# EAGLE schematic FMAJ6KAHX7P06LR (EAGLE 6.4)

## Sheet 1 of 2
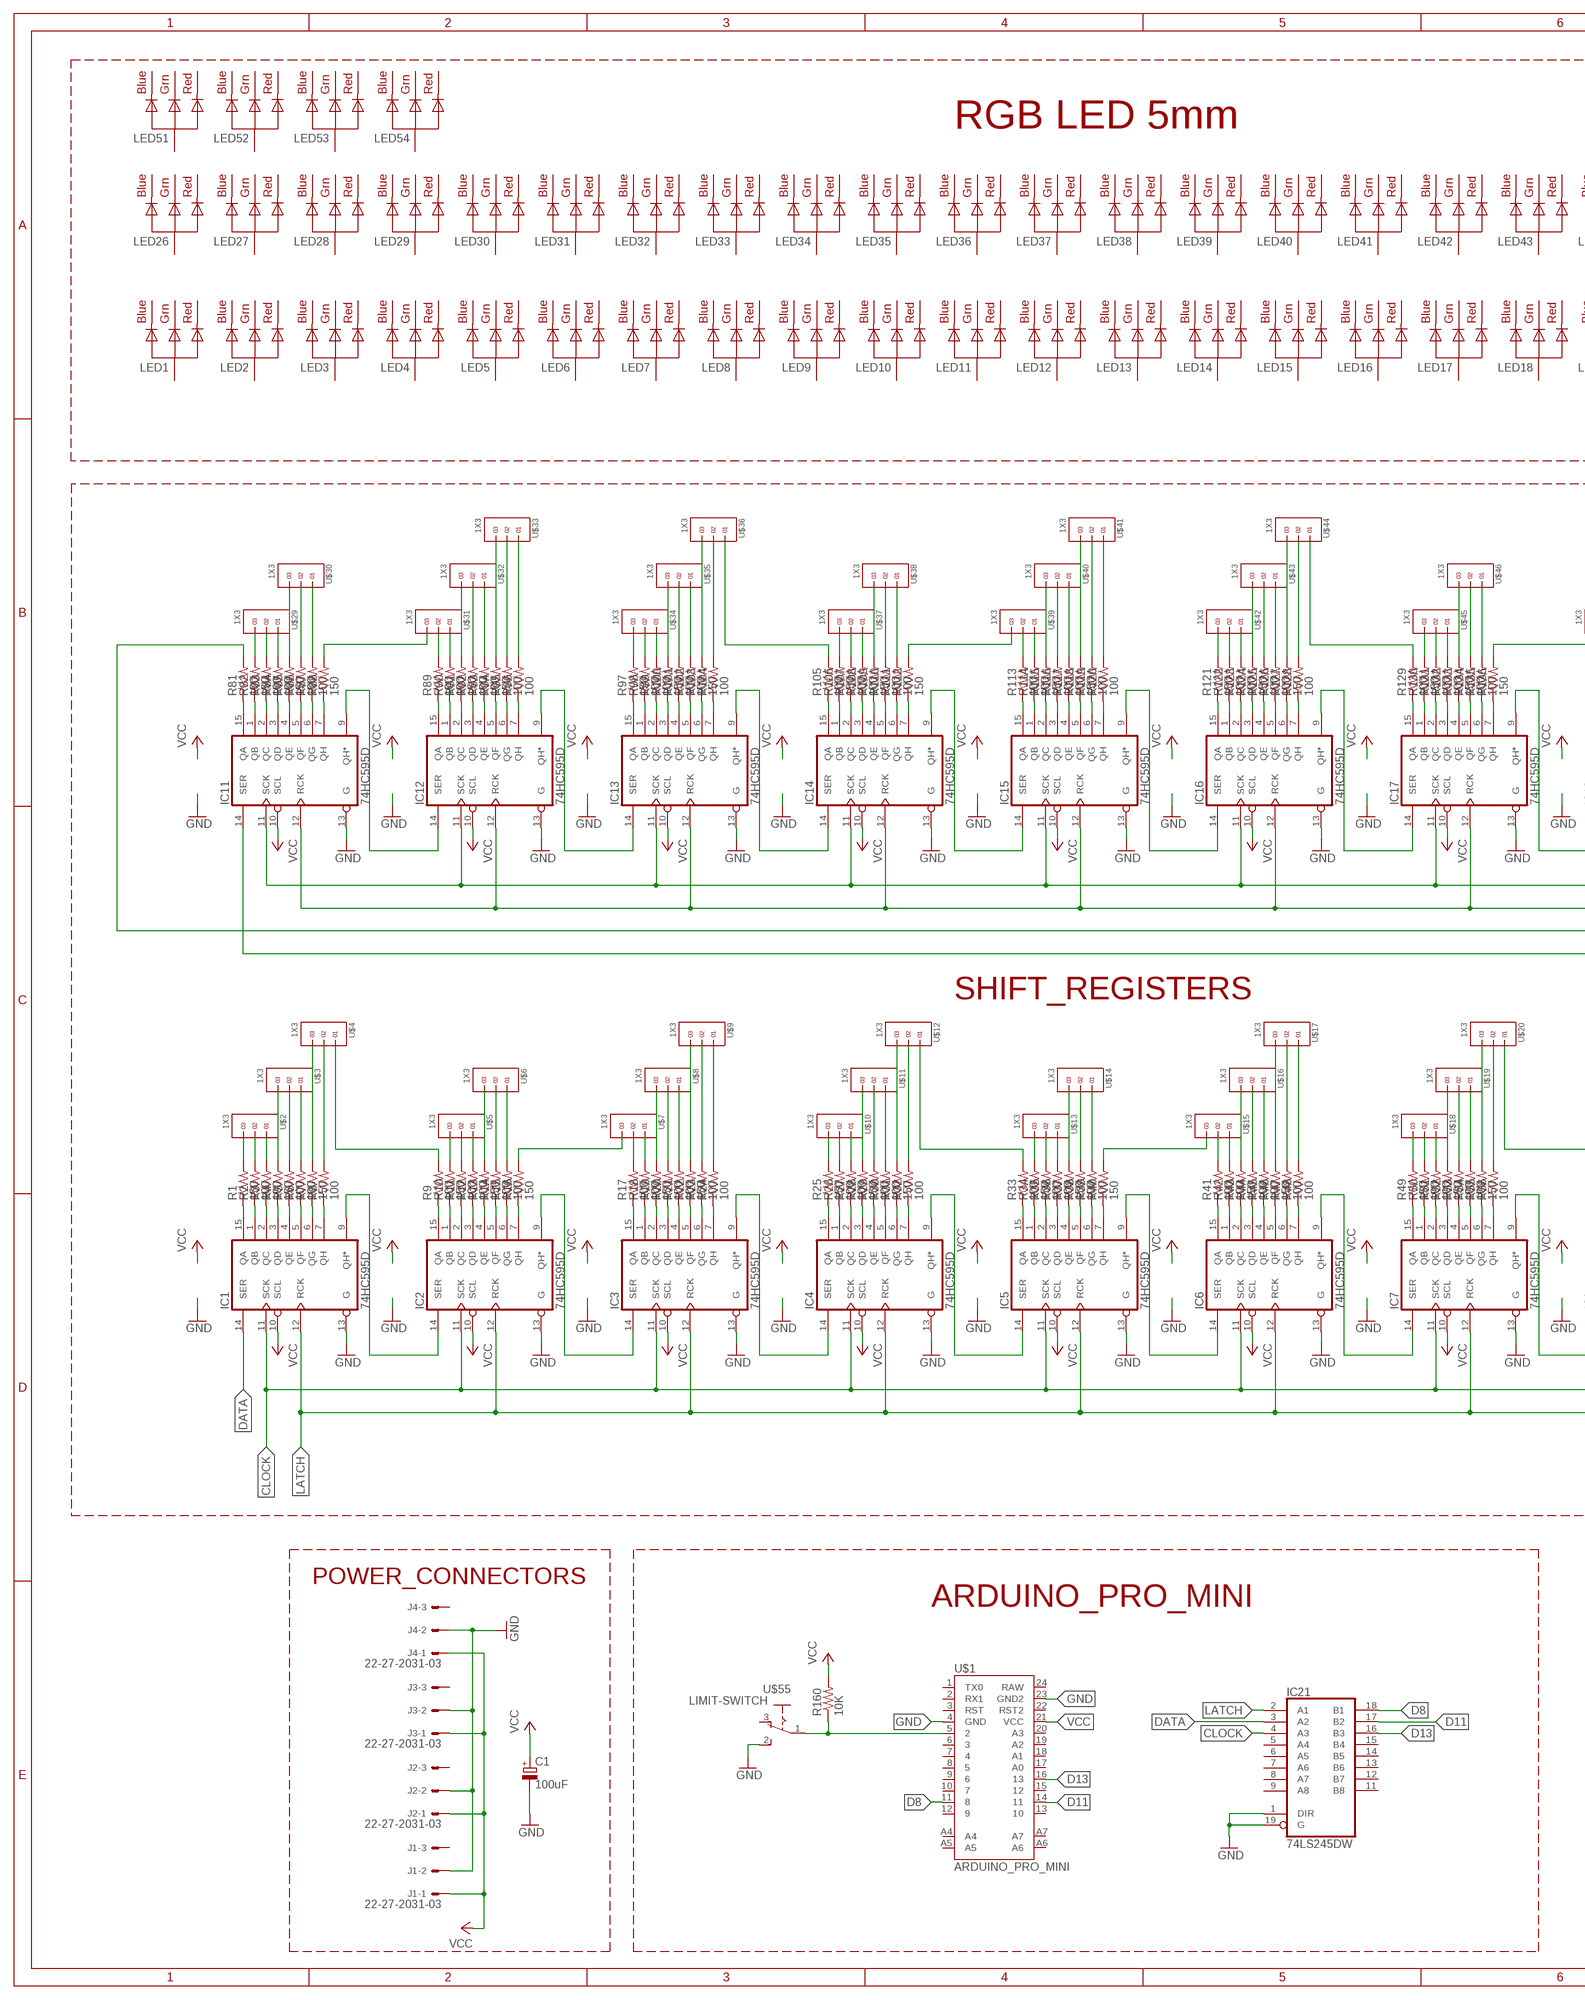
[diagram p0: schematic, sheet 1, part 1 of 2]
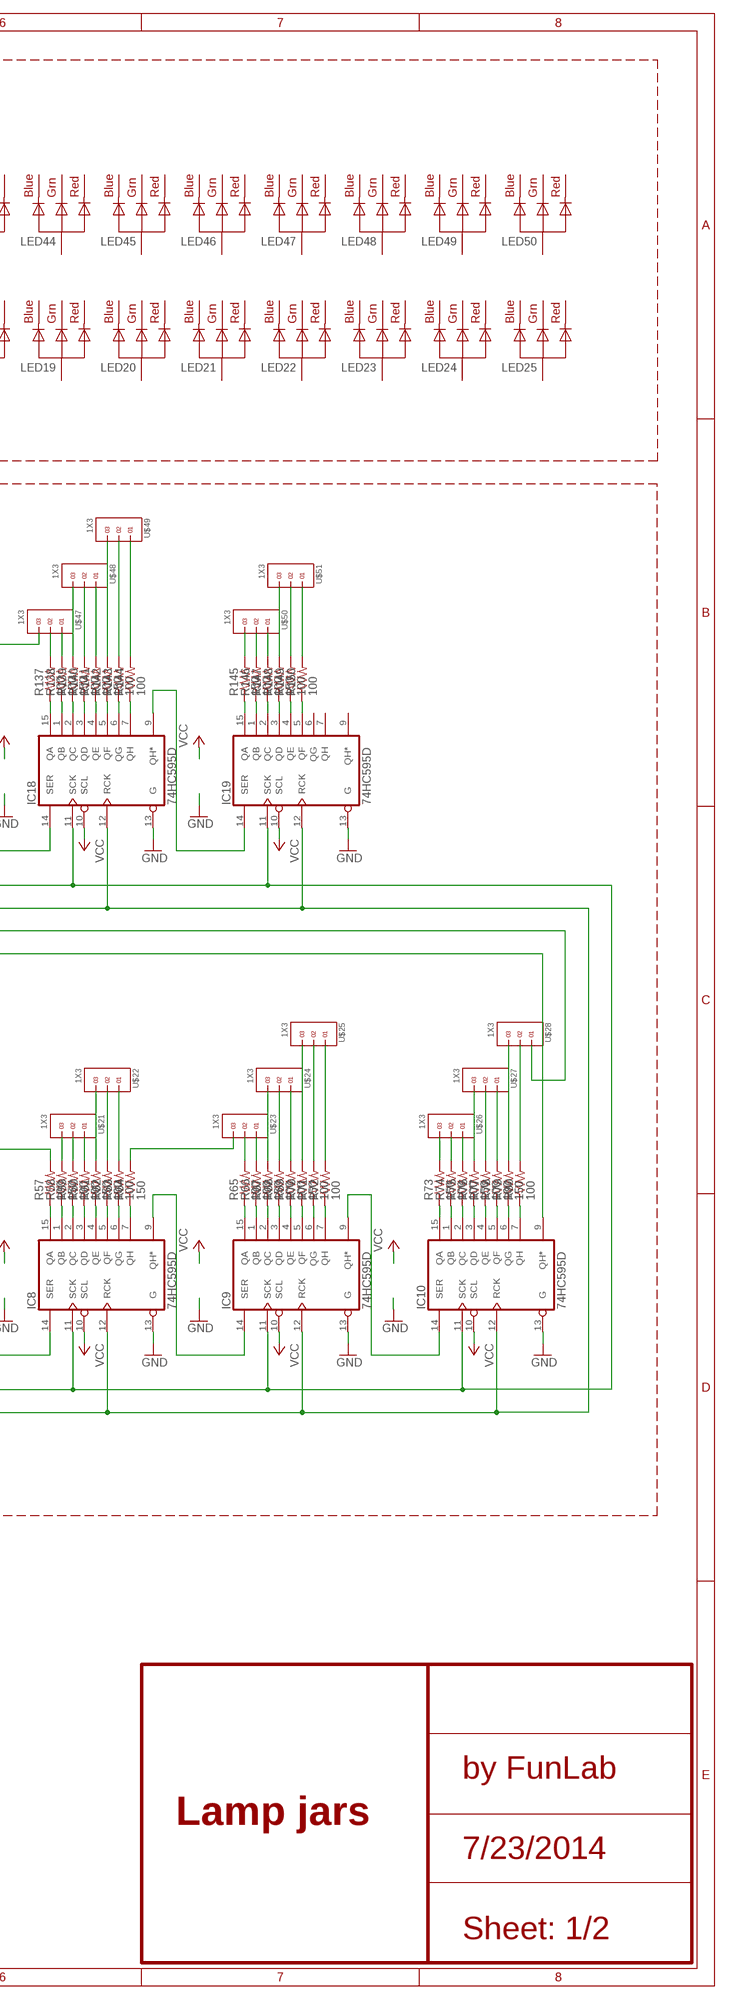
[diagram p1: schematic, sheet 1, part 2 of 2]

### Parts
C1  100uF  CPOL-EUE2.5-6  [E2,5-6]
IC1  74HC595D  [SO16]
IC2  74HC595D  [SO16]
IC3  74HC595D  [SO16]
IC4  74HC595D  [SO16]
IC5  74HC595D  [SO16]
IC6  74HC595D  [SO16]
IC7  74HC595D  [SO16]
IC8  74HC595D  [SO16]
IC9  74HC595D  [SO16]
IC10  74HC595D  [SO16]
IC11  74HC595D  [SO16]
IC12  74HC595D  [SO16]
IC13  74HC595D  [SO16]
IC14  74HC595D  [SO16]
IC15  74HC595D  [SO16]
IC16  74HC595D  [SO16]
IC17  74HC595D  [SO16]
IC18  74HC595D  [SO16]
IC19  74HC595D  [SO16]
IC21  74LS245DW  [SO20W]
J1  22-27-2031-03  [6410-03]
J2  22-27-2031-03  [6410-03]
J3  22-27-2031-03  [6410-03]
J4  22-27-2031-03  [6410-03]
LED1  RGBLED_CA-5MM  [LED5MMRGB]
LED2  RGBLED_CA-5MM  [LED5MMRGB]
LED3  RGBLED_CA-5MM  [LED5MMRGB]
LED4  RGBLED_CA-5MM  [LED5MMRGB]
LED5  RGBLED_CA-5MM  [LED5MMRGB]
LED6  RGBLED_CA-5MM  [LED5MMRGB]
LED7  RGBLED_CA-5MM  [LED5MMRGB]
LED8  RGBLED_CA-5MM  [LED5MMRGB]
LED9  RGBLED_CA-5MM  [LED5MMRGB]
LED10  RGBLED_CA-5MM  [LED5MMRGB]
LED11  RGBLED_CA-5MM  [LED5MMRGB]
LED12  RGBLED_CA-5MM  [LED5MMRGB]
LED13  RGBLED_CA-5MM  [LED5MMRGB]
LED14  RGBLED_CA-5MM  [LED5MMRGB]
LED15  RGBLED_CA-5MM  [LED5MMRGB]
LED16  RGBLED_CA-5MM  [LED5MMRGB]
LED17  RGBLED_CA-5MM  [LED5MMRGB]
LED18  RGBLED_CA-5MM  [LED5MMRGB]
LED19  RGBLED_CA-5MM  [LED5MMRGB]
LED20  RGBLED_CA-5MM  [LED5MMRGB]
LED21  RGBLED_CA-5MM  [LED5MMRGB]
LED22  RGBLED_CA-5MM  [LED5MMRGB]
LED23  RGBLED_CA-5MM  [LED5MMRGB]
LED24  RGBLED_CA-5MM  [LED5MMRGB]
LED25  RGBLED_CA-5MM  [LED5MMRGB]
LED26  RGBLED_CA-5MM  [LED5MMRGB]
LED27  RGBLED_CA-5MM  [LED5MMRGB]
LED28  RGBLED_CA-5MM  [LED5MMRGB]
LED29  RGBLED_CA-5MM  [LED5MMRGB]
LED30  RGBLED_CA-5MM  [LED5MMRGB]
LED31  RGBLED_CA-5MM  [LED5MMRGB]
LED32  RGBLED_CA-5MM  [LED5MMRGB]
LED33  RGBLED_CA-5MM  [LED5MMRGB]
LED34  RGBLED_CA-5MM  [LED5MMRGB]
LED35  RGBLED_CA-5MM  [LED5MMRGB]
LED36  RGBLED_CA-5MM  [LED5MMRGB]
LED37  RGBLED_CA-5MM  [LED5MMRGB]
LED38  RGBLED_CA-5MM  [LED5MMRGB]
LED39  RGBLED_CA-5MM  [LED5MMRGB]
LED40  RGBLED_CA-5MM  [LED5MMRGB]
LED41  RGBLED_CA-5MM  [LED5MMRGB]
LED42  RGBLED_CA-5MM  [LED5MMRGB]
LED43  RGBLED_CA-5MM  [LED5MMRGB]
LED44  RGBLED_CA-5MM  [LED5MMRGB]
LED45  RGBLED_CA-5MM  [LED5MMRGB]
LED46  RGBLED_CA-5MM  [LED5MMRGB]
LED47  RGBLED_CA-5MM  [LED5MMRGB]
LED48  RGBLED_CA-5MM  [LED5MMRGB]
LED49  RGBLED_CA-5MM  [LED5MMRGB]
LED50  RGBLED_CA-5MM  [LED5MMRGB]
LED51  RGBLED_CA-5MM  [LED5MMRGB]
LED52  RGBLED_CA-5MM  [LED5MMRGB]
LED53  RGBLED_CA-5MM  [LED5MMRGB]
LED54  RGBLED_CA-5MM  [LED5MMRGB]
R1  150  R-US_M0805  [M0805]
R2  100  R-US_M0805  [M0805]
R3  100  R-US_M0805  [M0805]
R4  150  R-US_M0805  [M0805]
R5  100  R-US_M0805  [M0805]
R6  100  R-US_M0805  [M0805]
R7  150  R-US_M0805  [M0805]
R8  100  R-US_M0805  [M0805]
R9  100  R-US_M0805  [M0805]
R10  150  R-US_M0805  [M0805]
R11  100  R-US_M0805  [M0805]
R12  100  R-US_M0805  [M0805]
R13  150  R-US_M0805  [M0805]
R14  100  R-US_M0805  [M0805]
R15  100  R-US_M0805  [M0805]
R16  150  R-US_M0805  [M0805]
R17  100  R-US_M0805  [M0805]
R18  100  R-US_M0805  [M0805]
R19  150  R-US_M0805  [M0805]
R20  100  R-US_M0805  [M0805]
R21  100  R-US_M0805  [M0805]
R22  150  R-US_M0805  [M0805]
R23  100  R-US_M0805  [M0805]
R24  100  R-US_M0805  [M0805]
R25  150  R-US_M0805  [M0805]
R26  100  R-US_M0805  [M0805]
R27  100  R-US_M0805  [M0805]
R28  150  R-US_M0805  [M0805]
R29  100  R-US_M0805  [M0805]
R30  100  R-US_M0805  [M0805]
R31  150  R-US_M0805  [M0805]
R32  100  R-US_M0805  [M0805]
R33  100  R-US_M0805  [M0805]
R34  150  R-US_M0805  [M0805]
R35  100  R-US_M0805  [M0805]
R36  100  R-US_M0805  [M0805]
R37  150  R-US_M0805  [M0805]
R38  100  R-US_M0805  [M0805]
R39  100  R-US_M0805  [M0805]
R40  150  R-US_M0805  [M0805]
R41  100  R-US_M0805  [M0805]
R42  100  R-US_M0805  [M0805]
R43  150  R-US_M0805  [M0805]
R44  100  R-US_M0805  [M0805]
R45  100  R-US_M0805  [M0805]
R46  150  R-US_M0805  [M0805]
R47  100  R-US_M0805  [M0805]
R48  100  R-US_M0805  [M0805]
R49  150  R-US_M0805  [M0805]
R50  100  R-US_M0805  [M0805]
R51  100  R-US_M0805  [M0805]
R52  150  R-US_M0805  [M0805]
R53  100  R-US_M0805  [M0805]
R54  100  R-US_M0805  [M0805]
R55  150  R-US_M0805  [M0805]
R56  100  R-US_M0805  [M0805]
R57  100  R-US_M0805  [M0805]
R58  150  R-US_M0805  [M0805]
R59  100  R-US_M0805  [M0805]
R60  100  R-US_M0805  [M0805]
R61  150  R-US_M0805  [M0805]
R62  100  R-US_M0805  [M0805]
R63  100  R-US_M0805  [M0805]
R64  150  R-US_M0805  [M0805]
R65  100  R-US_M0805  [M0805]
R66  100  R-US_M0805  [M0805]
R67  150  R-US_M0805  [M0805]
R68  100  R-US_M0805  [M0805]
R69  100  R-US_M0805  [M0805]
R70  150  R-US_M0805  [M0805]
R71  100  R-US_M0805  [M0805]
R72  100  R-US_M0805  [M0805]
R73  150  R-US_M0805  [M0805]
R74  100  R-US_M0805  [M0805]
R75  100  R-US_M0805  [M0805]
R76  150  R-US_M0805  [M0805]
R77  100  R-US_M0805  [M0805]
R78  100  R-US_M0805  [M0805]
R79  150  R-US_M0805  [M0805]
R80  100  R-US_M0805  [M0805]
R81  100  R-US_M0805  [M0805]
R82  150  R-US_M0805  [M0805]
R83  100  R-US_M0805  [M0805]
R84  100  R-US_M0805  [M0805]
R85  150  R-US_M0805  [M0805]
R86  100  R-US_M0805  [M0805]
R87  100  R-US_M0805  [M0805]
R88  150  R-US_M0805  [M0805]
R89  100  R-US_M0805  [M0805]
R90  100  R-US_M0805  [M0805]
R91  150  R-US_M0805  [M0805]
R92  100  R-US_M0805  [M0805]
R93  100  R-US_M0805  [M0805]
R94  150  R-US_M0805  [M0805]
R95  100  R-US_M0805  [M0805]
R96  100  R-US_M0805  [M0805]
R97  150  R-US_M0805  [M0805]
R98  100  R-US_M0805  [M0805]
R99  100  R-US_M0805  [M0805]
R100  150  R-US_M0805  [M0805]
R101  100  R-US_M0805  [M0805]
R102  100  R-US_M0805  [M0805]
R103  150  R-US_M0805  [M0805]
R104  100  R-US_M0805  [M0805]
R105  100  R-US_M0805  [M0805]
R106  150  R-US_M0805  [M0805]
R107  100  R-US_M0805  [M0805]
R108  100  R-US_M0805  [M0805]
R109  150  R-US_M0805  [M0805]
R110  100  R-US_M0805  [M0805]
R111  100  R-US_M0805  [M0805]
R112  150  R-US_M0805  [M0805]
R113  100  R-US_M0805  [M0805]
R114  100  R-US_M0805  [M0805]
R115  150  R-US_M0805  [M0805]
R116  100  R-US_M0805  [M0805]
R117  100  R-US_M0805  [M0805]
R118  150  R-US_M0805  [M0805]
R119  100  R-US_M0805  [M0805]
R120  100  R-US_M0805  [M0805]
R121  150  R-US_M0805  [M0805]
R122  100  R-US_M0805  [M0805]
R123  100  R-US_M0805  [M0805]
R124  150  R-US_M0805  [M0805]
R125  100  R-US_M0805  [M0805]
R126  100  R-US_M0805  [M0805]
R127  150  R-US_M0805  [M0805]
R128  100  R-US_M0805  [M0805]
R129  100  R-US_M0805  [M0805]
R130  150  R-US_M0805  [M0805]
R131  100  R-US_M0805  [M0805]
R132  100  R-US_M0805  [M0805]
R133  150  R-US_M0805  [M0805]
R134  100  R-US_M0805  [M0805]
R135  100  R-US_M0805  [M0805]
R136  150  R-US_M0805  [M0805]
R137  100  R-US_M0805  [M0805]
R138  100  R-US_M0805  [M0805]
R139  150  R-US_M0805  [M0805]
R140  100  R-US_M0805  [M0805]
R141  100  R-US_M0805  [M0805]
R142  150  R-US_M0805  [M0805]
R143  100  R-US_M0805  [M0805]
R144  100  R-US_M0805  [M0805]
R145  150  R-US_M0805  [M0805]
R146  100  R-US_M0805  [M0805]
R147  100  R-US_M0805  [M0805]
R148  150  R-US_M0805  [M0805]
R149  100  R-US_M0805  [M0805]
R150  100  R-US_M0805  [M0805]
R160  10K  R-US_0207/10  [0207/10]
U$1  ARDUINO_PRO_MINI  [ARDUINO_PRO_MINI]
U$2  1X3  [1X3]
U$3  1X3  [1X3]
U$4  1X3  [1X3]
U$5  1X3  [1X3]
U$6  1X3  [1X3]
U$7  1X3  [1X3]
U$8  1X3  [1X3]
U$9  1X3  [1X3]
U$10  1X3  [1X3]
U$11  1X3  [1X3]
U$12  1X3  [1X3]
U$13  1X3  [1X3]
U$14  1X3  [1X3]
U$15  1X3  [1X3]
U$16  1X3  [1X3]
U$17  1X3  [1X3]
U$18  1X3  [1X3]
U$19  1X3  [1X3]
U$20  1X3  [1X3]
U$21  1X3  [1X3]
U$22  1X3  [1X3]
U$23  1X3  [1X3]
U$24  1X3  [1X3]
U$25  1X3  [1X3]
U$26  1X3  [1X3]
U$27  1X3  [1X3]
U$28  1X3  [1X3]
U$29  1X3  [1X3]
U$30  1X3  [1X3]
U$31  1X3  [1X3]
U$32  1X3  [1X3]
U$33  1X3  [1X3]
U$34  1X3  [1X3]
U$35  1X3  [1X3]
U$36  1X3  [1X3]
U$37  1X3  [1X3]
U$38  1X3  [1X3]
U$39  1X3  [1X3]
U$40  1X3  [1X3]
U$41  1X3  [1X3]
U$42  1X3  [1X3]
U$43  1X3  [1X3]
U$44  1X3  [1X3]
U$45  1X3  [1X3]
U$46  1X3  [1X3]
U$47  1X3  [1X3]
U$48  1X3  [1X3]
U$49  1X3  [1X3]
U$50  1X3  [1X3]
U$51  1X3  [1X3]
U$55  LIMIT-SWITCH  [LIMIT-SWITCH]

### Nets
CLOCK: IC1.11(SCK) IC2.11(SCK) IC3.11(SCK) IC4.11(SCK) IC5.11(SCK) IC6.11(SCK) IC7.11(SCK) IC8.11(SCK) IC9.11(SCK) IC10.11(SCK) IC11.11(SCK) IC12.11(SCK) IC13.11(SCK) IC14.11(SCK) IC15.11(SCK) IC16.11(SCK) IC17.11(SCK) IC18.11(SCK) IC19.11(SCK) IC21.4(A3)
D8: IC21.18(B1) U$1.11
D11: IC21.17(B2) U$1.14
D13: IC21.16(B3) U$1.16
DATA: IC1.14(SER) IC21.3(A2)
GND: C1.- IC1.13(G) IC2.13(G) IC3.13(G) IC4.13(G) IC5.13(G) IC6.13(G) IC7.13(G) IC8.13(G) IC9.13(G) IC10.13(G) IC11.13(G) IC12.13(G) IC13.13(G) IC14.13(G) IC15.13(G) IC16.13(G) IC17.13(G) IC18.13(G) IC19.13(G) IC21.1(DIR) IC21.19(G) J1.2 J2.2 J3.2 J4.2 U$1.4(GND) U$1.23(GND2) U$55.2(S) ; also sheet 2
LATCH: IC1.12(RCK) IC2.12(RCK) IC3.12(RCK) IC4.12(RCK) IC5.12(RCK) IC6.12(RCK) IC7.12(RCK) IC8.12(RCK) IC9.12(RCK) IC10.12(RCK) IC11.12(RCK) IC12.12(RCK) IC13.12(RCK) IC14.12(RCK) IC15.12(RCK) IC16.12(RCK) IC17.12(RCK) IC18.12(RCK) IC19.12(RCK) IC21.2(A1)
N$1: R160.1 U$1.5 U$55.1(P)
N$5: R81.2 U$28.1
N$6: IC10.9(QH*) IC11.14(SER)
N$29: IC1.15(QA) R1.1
N$30: IC1.1(QB) R2.1
N$31: IC1.2(QC) R3.1
N$32: R1.2 U$2.3
N$33: R2.2 U$2.2
N$34: R3.2 U$2.1
N$35: R4.2 U$3.3
N$36: R5.2 U$3.2
N$37: R6.2 U$3.1
N$38: R7.2 U$4.3
N$39: R8.2 U$4.2
N$40: IC1.3(QD) R4.1
N$41: IC1.4(QE) R5.1
N$42: IC1.5(QF) R6.1
N$43: IC1.6(QG) R7.1
N$44: IC1.7(QH) R8.1
N$45: IC2.15(QA) R9.1
N$46: R9.2 U$4.1
N$47: R10.2 U$5.3
N$48: R11.2 U$5.2
N$49: R12.2 U$5.1
N$50: R13.2 U$6.3
N$51: R14.2 U$6.2
N$52: R15.2 U$6.1
N$53: R16.2 U$7.3
N$54: R17.2 U$7.2
N$55: R18.2 U$7.1
N$56: R19.2 U$8.3
N$57: R20.2 U$8.2
N$58: R21.2 U$8.1
N$59: R22.2 U$9.3
N$60: R23.2 U$9.2
N$61: R24.2 U$9.1
N$62: R25.2 U$10.3
N$63: R26.2 U$10.2
N$64: R27.2 U$10.1
N$65: R28.2 U$11.3
N$66: R29.2 U$11.2
N$67: R30.2 U$11.1
N$68: R31.2 U$12.3
N$69: R32.2 U$12.2
N$70: R33.2 U$12.1
N$71: R34.2 U$13.3
N$72: R35.2 U$13.2
N$73: R36.2 U$13.1
N$74: R37.2 U$14.3
N$75: R38.2 U$14.2
N$76: R39.2 U$14.1
N$77: R40.2 U$15.3
N$78: R41.2 U$15.2
N$79: R42.2 U$15.1
N$80: R43.2 U$16.3
N$81: R44.2 U$16.2
N$82: R45.2 U$16.1
N$83: R46.2 U$17.3
N$84: R47.2 U$17.2
N$85: R48.2 U$17.1
N$86: R49.2 U$18.3
N$87: R50.2 U$18.2
N$88: R51.2 U$18.1
N$89: R52.2 U$19.3
N$90: R53.2 U$19.2
N$91: R54.2 U$19.1
N$92: R55.2 U$20.3
N$93: R56.2 U$20.2
N$94: R57.2 U$20.1
N$95: R58.2 U$21.3
N$96: R59.2 U$21.2
N$97: R60.2 U$21.1
N$98: R61.2 U$22.3
N$99: R62.2 U$22.2
N$100: R63.2 U$22.1
N$101: R64.2 U$23.3
N$102: R65.2 U$23.2
N$103: R66.2 U$23.1
N$104: R67.2 U$24.3
N$105: R68.2 U$24.2
N$106: R69.2 U$24.1
N$107: R70.2 U$25.3
N$108: R71.2 U$25.2
N$109: R72.2 U$25.1
N$110: R73.2 U$26.3
N$111: R74.2 U$26.2
N$112: R75.2 U$26.1
N$113: R76.2 U$27.3
N$114: R77.2 U$27.2
N$115: R78.2 U$27.1
N$116: R79.2 U$28.3
N$117: R80.2 U$28.2
N$118: R82.2 U$29.3
N$119: R83.2 U$29.2
N$120: R84.2 U$29.1
N$121: R85.2 U$30.3
N$122: R86.2 U$30.2
N$123: R87.2 U$30.1
N$124: R88.2 U$31.3
N$125: R89.2 U$31.2
N$126: R90.2 U$31.1
N$127: R91.2 U$32.3
N$128: R92.2 U$32.2
N$129: R93.2 U$32.1
N$130: R94.2 U$33.3
N$131: R95.2 U$33.2
N$132: R96.2 U$33.1
N$133: R97.2 U$34.3
N$134: R98.2 U$34.2
N$135: R99.2 U$34.1
N$136: R100.2 U$35.3
N$137: R101.2 U$35.2
N$138: R102.2 U$35.1
N$139: R103.2 U$36.3
N$140: R104.2 U$36.2
N$141: R105.2 U$36.1
N$142: R106.2 U$37.3
N$143: R107.2 U$37.2
N$144: R108.2 U$37.1
N$145: R109.2 U$38.3
N$146: R110.2 U$38.2
N$147: R111.2 U$38.1
N$148: R112.2 U$39.3
N$149: R113.2 U$39.2
N$150: R114.2 U$39.1
N$151: R115.2 U$40.3
N$152: R116.2 U$40.2
N$153: R117.2 U$40.1
N$154: R118.2 U$41.3
N$155: R119.2 U$41.2
N$156: R120.2 U$41.1
N$157: R121.2 U$42.3
N$158: R122.2 U$42.2
N$159: R123.2 U$42.1
N$160: R124.2 U$43.3
N$161: R125.2 U$43.2
N$162: R126.2 U$43.1
N$163: R127.2 U$44.3
N$164: R128.2 U$44.2
N$165: R129.2 U$44.1
N$166: R130.2 U$45.3
N$167: R131.2 U$45.2
N$168: R132.2 U$45.1
N$169: R133.2 U$46.3
N$170: R134.2 U$46.2
N$171: R135.2 U$46.1
N$172: R136.2 U$47.3
N$173: R137.2 U$47.2
N$174: R138.2 U$47.1
N$175: R139.2 U$48.3
N$176: R140.2 U$48.2
N$177: R141.2 U$48.1
N$178: R142.2 U$49.3
N$179: R143.2 U$49.2
N$180: R144.2 U$49.1
N$181: R145.2 U$50.3
N$182: R146.2 U$50.2
N$183: R147.2 U$50.1
N$184: R148.2 U$51.3
N$185: R149.2 U$51.2
N$186: R150.2 U$51.1
N$196: IC11.15(QA) R81.1
N$197: IC11.1(QB) R82.1
N$198: IC11.2(QC) R83.1
N$199: IC11.3(QD) R84.1
N$200: IC11.4(QE) R85.1
N$201: IC11.5(QF) R86.1
N$202: IC11.6(QG) R87.1
N$203: IC11.7(QH) R88.1
N$204: IC12.15(QA) R89.1
N$205: IC12.1(QB) R90.1
N$206: IC12.2(QC) R91.1
N$207: IC12.3(QD) R92.1
N$208: IC12.4(QE) R93.1
N$209: IC12.5(QF) R94.1
N$210: IC12.6(QG) R95.1
N$211: IC12.7(QH) R96.1
N$212: IC13.15(QA) R97.1
N$213: IC13.1(QB) R98.1
N$214: IC13.2(QC) R99.1
N$215: IC13.3(QD) R100.1
N$216: IC13.4(QE) R101.1
N$217: IC13.5(QF) R102.1
N$218: IC13.6(QG) R103.1
N$219: IC13.7(QH) R104.1
N$220: IC14.15(QA) R105.1
N$221: IC14.1(QB) R106.1
N$222: IC14.2(QC) R107.1
N$223: IC14.3(QD) R108.1
N$224: IC14.4(QE) R109.1
N$225: IC14.5(QF) R110.1
N$226: IC14.6(QG) R111.1
N$227: IC14.7(QH) R112.1
N$228: IC15.15(QA) R113.1
N$229: IC15.1(QB) R114.1
N$230: IC15.2(QC) R115.1
N$231: IC15.3(QD) R116.1
N$232: IC15.4(QE) R117.1
N$233: IC15.5(QF) R118.1
N$234: IC15.6(QG) R119.1
N$235: IC15.7(QH) R120.1
N$236: IC16.15(QA) R121.1
N$237: IC16.1(QB) R122.1
N$238: IC16.2(QC) R123.1
N$239: IC16.3(QD) R124.1
N$240: IC16.4(QE) R125.1
N$241: IC16.5(QF) R126.1
N$242: IC16.6(QG) R127.1
N$243: IC16.7(QH) R128.1
N$244: IC17.15(QA) R129.1
N$245: IC17.1(QB) R130.1
N$246: IC17.2(QC) R131.1
N$247: IC17.3(QD) R132.1
N$248: IC17.4(QE) R133.1
N$249: IC17.5(QF) R134.1
N$250: IC17.6(QG) R135.1
N$251: IC17.7(QH) R136.1
N$252: IC18.15(QA) R137.1
N$253: IC18.1(QB) R138.1
N$254: IC18.2(QC) R139.1
N$255: IC18.3(QD) R140.1
N$256: IC18.4(QE) R141.1
N$257: IC18.5(QF) R142.1
N$258: IC18.6(QG) R143.1
N$259: IC18.7(QH) R144.1
N$260: IC19.15(QA) R145.1
N$261: IC19.1(QB) R146.1
N$262: IC19.2(QC) R147.1
N$263: IC19.3(QD) R148.1
N$264: IC19.4(QE) R149.1
N$265: IC19.5(QF) R150.1
N$276: IC10.7(QH) R80.1
N$277: IC10.6(QG) R79.1
N$278: IC10.5(QF) R78.1
N$279: IC10.4(QE) R77.1
N$280: IC10.3(QD) R76.1
N$281: IC10.2(QC) R75.1
N$282: IC10.1(QB) R74.1
N$283: IC10.15(QA) R73.1
N$284: IC9.7(QH) R72.1
N$285: IC9.6(QG) R71.1
N$286: IC9.5(QF) R70.1
N$287: IC9.4(QE) R69.1
N$288: IC9.3(QD) R68.1
N$289: IC9.2(QC) R67.1
N$290: IC9.1(QB) R66.1
N$291: IC9.15(QA) R65.1
N$292: IC8.7(QH) R64.1
N$293: IC8.6(QG) R63.1
N$294: IC8.5(QF) R62.1
N$295: IC8.4(QE) R61.1
N$296: IC8.3(QD) R60.1
N$297: IC8.2(QC) R59.1
N$298: IC8.1(QB) R58.1
N$299: IC8.15(QA) R57.1
N$300: IC7.7(QH) R56.1
N$301: IC7.6(QG) R55.1
N$302: IC7.5(QF) R54.1
N$303: IC7.4(QE) R53.1
N$304: IC7.3(QD) R52.1
N$305: IC7.2(QC) R51.1
N$306: IC7.1(QB) R50.1
N$307: IC7.15(QA) R49.1
N$308: IC6.7(QH) R48.1
N$309: IC6.6(QG) R47.1
N$310: IC6.5(QF) R46.1
N$311: IC6.4(QE) R45.1
N$312: IC6.3(QD) R44.1
N$313: IC6.2(QC) R43.1
N$314: IC6.1(QB) R42.1
N$315: IC6.15(QA) R41.1
N$316: IC5.7(QH) R40.1
N$317: IC5.6(QG) R39.1
N$318: IC5.5(QF) R38.1
N$319: IC5.4(QE) R37.1
N$320: IC5.3(QD) R36.1
N$321: IC5.2(QC) R35.1
N$322: IC5.1(QB) R34.1
N$323: IC5.15(QA) R33.1
N$324: IC4.7(QH) R32.1
N$325: IC4.6(QG) R31.1
N$326: IC4.5(QF) R30.1
N$327: IC4.4(QE) R29.1
N$328: IC4.3(QD) R28.1
N$329: IC4.2(QC) R27.1
N$330: IC4.1(QB) R26.1
N$331: IC4.15(QA) R25.1
N$332: IC3.7(QH) R24.1
N$333: IC3.6(QG) R23.1
N$334: IC3.5(QF) R22.1
N$335: IC3.4(QE) R21.1
N$336: IC3.3(QD) R20.1
N$337: IC3.2(QC) R19.1
N$338: IC3.1(QB) R18.1
N$339: IC3.15(QA) R17.1
N$340: IC2.7(QH) R16.1
N$341: IC2.6(QG) R15.1
N$342: IC2.5(QF) R14.1
N$343: IC2.4(QE) R13.1
N$344: IC2.3(QD) R12.1
N$345: IC2.2(QC) R11.1
N$346: IC2.1(QB) R10.1
N$347: IC2.9(QH*) IC3.14(SER)
N$348: IC1.9(QH*) IC2.14(SER)
N$349: IC3.9(QH*) IC4.14(SER)
N$350: IC4.9(QH*) IC5.14(SER)
N$351: IC5.9(QH*) IC6.14(SER)
N$352: IC6.9(QH*) IC7.14(SER)
N$353: IC7.9(QH*) IC8.14(SER)
N$354: IC8.9(QH*) IC9.14(SER)
N$355: IC9.9(QH*) IC10.14(SER)
N$356: IC11.9(QH*) IC12.14(SER)
N$357: IC12.9(QH*) IC13.14(SER)
N$358: IC13.9(QH*) IC14.14(SER)
N$359: IC14.9(QH*) IC15.14(SER)
N$360: IC15.9(QH*) IC16.14(SER)
N$361: IC16.9(QH*) IC17.14(SER)
N$362: IC17.9(QH*) IC18.14(SER)
N$363: IC18.9(QH*) IC19.14(SER)
VCC: C1.+ IC1.10(SCL) IC2.10(SCL) IC3.10(SCL) IC4.10(SCL) IC5.10(SCL) IC6.10(SCL) IC7.10(SCL) IC8.10(SCL) IC9.10(SCL) IC10.10(SCL) IC11.10(SCL) IC12.10(SCL) IC13.10(SCL) IC14.10(SCL) IC15.10(SCL) IC16.10(SCL) IC17.10(SCL) IC18.10(SCL) IC19.10(SCL) J1.1 J2.1 J3.1 J4.1 R160.2 U$1.21(VCC) ; also sheet 2
Unconnected: IC19.6(QG) IC19.7(QH) IC19.9(QH*) IC21.5(A4) IC21.6(A5) IC21.7(A6) IC21.8(A7) IC21.9(A8) IC21.11(B8) IC21.12(B7) IC21.13(B6) IC21.14(B5) IC21.15(B4) J1.3 J2.3 J3.3 J4.3 LED1.1(RED) LED1.2(VCC) LED1.3(GREEN) LED1.4(BLUE) LED2.1(RED) LED2.2(VCC) LED2.3(GREEN) LED2.4(BLUE) LED3.1(RED) LED3.2(VCC) LED3.3(GREEN) LED3.4(BLUE) LED4.1(RED) LED4.2(VCC) LED4.3(GREEN) LED4.4(BLUE) LED5.1(RED) LED5.2(VCC) LED5.3(GREEN) LED5.4(BLUE) LED6.1(RED) LED6.2(VCC) LED6.3(GREEN) LED6.4(BLUE) LED7.1(RED) LED7.2(VCC) LED7.3(GREEN) LED7.4(BLUE) LED8.1(RED) LED8.2(VCC) LED8.3(GREEN) LED8.4(BLUE) LED9.1(RED) LED9.2(VCC) LED9.3(GREEN) LED9.4(BLUE) LED10.1(RED) LED10.2(VCC) LED10.3(GREEN) LED10.4(BLUE) LED11.1(RED) LED11.2(VCC) LED11.3(GREEN) LED11.4(BLUE) LED12.1(RED) LED12.2(VCC) LED12.3(GREEN) LED12.4(BLUE) LED13.1(RED) LED13.2(VCC) LED13.3(GREEN) LED13.4(BLUE) LED14.1(RED) LED14.2(VCC) LED14.3(GREEN) LED14.4(BLUE) LED15.1(RED) LED15.2(VCC) LED15.3(GREEN) LED15.4(BLUE) LED16.1(RED) LED16.2(VCC) LED16.3(GREEN) LED16.4(BLUE) LED17.1(RED) LED17.2(VCC) LED17.3(GREEN) LED17.4(BLUE) LED18.1(RED) LED18.2(VCC) LED18.3(GREEN) LED18.4(BLUE) LED19.1(RED) LED19.2(VCC) LED19.3(GREEN) LED19.4(BLUE) LED20.1(RED) LED20.2(VCC) LED20.3(GREEN) LED20.4(BLUE) LED21.1(RED) LED21.2(VCC) LED21.3(GREEN) LED21.4(BLUE) LED22.1(RED) LED22.2(VCC) LED22.3(GREEN) LED22.4(BLUE) LED23.1(RED) LED23.2(VCC) LED23.3(GREEN) LED23.4(BLUE) LED24.1(RED) LED24.2(VCC) LED24.3(GREEN) LED24.4(BLUE) LED25.1(RED) LED25.2(VCC) LED25.3(GREEN) LED25.4(BLUE) LED26.1(RED) LED26.2(VCC) LED26.3(GREEN) LED26.4(BLUE) LED27.1(RED) LED27.2(VCC) LED27.3(GREEN) LED27.4(BLUE) LED28.1(RED) LED28.2(VCC) LED28.3(GREEN) LED28.4(BLUE) LED29.1(RED) LED29.2(VCC) LED29.3(GREEN) LED29.4(BLUE) LED30.1(RED) LED30.2(VCC) LED30.3(GREEN) LED30.4(BLUE) LED31.1(RED) LED31.2(VCC) LED31.3(GREEN) LED31.4(BLUE) LED32.1(RED) LED32.2(VCC) LED32.3(GREEN) LED32.4(BLUE) LED33.1(RED) LED33.2(VCC) LED33.3(GREEN) LED33.4(BLUE) LED34.1(RED) LED34.2(VCC) LED34.3(GREEN) LED34.4(BLUE) LED35.1(RED) LED35.2(VCC) LED35.3(GREEN) LED35.4(BLUE) LED36.1(RED) LED36.2(VCC) LED36.3(GREEN) LED36.4(BLUE) LED37.1(RED) LED37.2(VCC) LED37.3(GREEN) LED37.4(BLUE) LED38.1(RED) LED38.2(VCC) LED38.3(GREEN) LED38.4(BLUE) LED39.1(RED) LED39.2(VCC) LED39.3(GREEN) LED39.4(BLUE) LED40.1(RED) LED40.2(VCC) LED40.3(GREEN) LED40.4(BLUE) LED41.1(RED) LED41.2(VCC) LED41.3(GREEN) LED41.4(BLUE) LED42.1(RED) LED42.2(VCC) LED42.3(GREEN) LED42.4(BLUE) LED43.1(RED) LED43.2(VCC) LED43.3(GREEN) LED43.4(BLUE) LED44.1(RED) LED44.2(VCC) LED44.3(GREEN) LED44.4(BLUE) LED45.1(RED) LED45.2(VCC) LED45.3(GREEN) LED45.4(BLUE) LED46.1(RED) LED46.2(VCC) LED46.3(GREEN) LED46.4(BLUE) LED47.1(RED) LED47.2(VCC) LED47.3(GREEN) LED47.4(BLUE) LED48.1(RED) LED48.2(VCC) LED48.3(GREEN) LED48.4(BLUE) LED49.1(RED) LED49.2(VCC) LED49.3(GREEN) LED49.4(BLUE) LED50.1(RED) LED50.2(VCC) LED50.3(GREEN) LED50.4(BLUE) LED51.1(RED) LED51.2(VCC) LED51.3(GREEN) LED51.4(BLUE) LED52.1(RED) LED52.2(VCC) LED52.3(GREEN) LED52.4(BLUE) LED53.1(RED) LED53.2(VCC) LED53.3(GREEN) LED53.4(BLUE) LED54.1(RED) LED54.2(VCC) LED54.3(GREEN) LED54.4(BLUE) U$1.1(TX0) U$1.2(RX1) U$1.3(RST) U$1.6 U$1.7 U$1.8 U$1.9 U$1.10 U$1.12 U$1.13 U$1.15 U$1.17(A0) U$1.18(A1) U$1.19(A2) U$1.20(A3) U$1.22(RST2) U$1.24(RAW) U$1.A4 U$1.A5 U$1.A6 U$1.A7 U$55.3(O)

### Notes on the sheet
- RGB LED 5mm
- SHIFT_REGISTERS
- POWER_CONNECTORS
- ARDUINO_PRO_MINI
- by FunLab
- Lamp jars
- 7/23/2014
- Sheet: 1/2

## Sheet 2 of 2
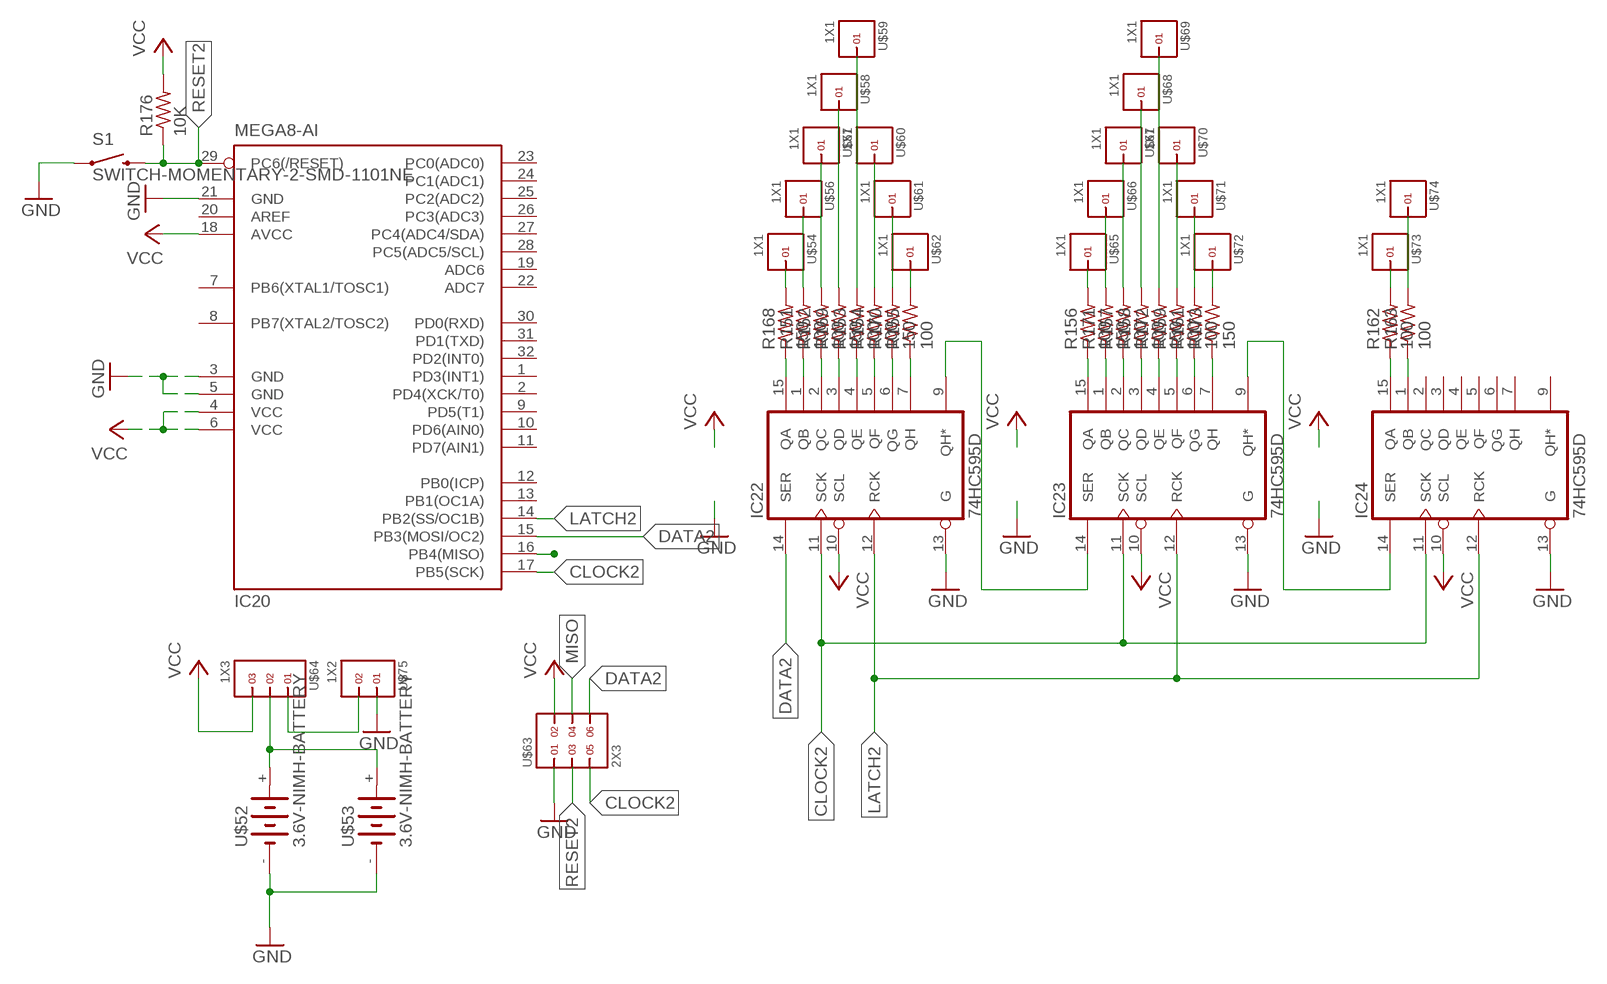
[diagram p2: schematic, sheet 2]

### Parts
IC20  MEGA8-AI  [TQFP32-08]
IC22  74HC595D  [SO16]
IC23  74HC595D  [SO16]
IC24  74HC595D  [SO16]
R151  100  R-US_M0805  [M0805]
R152  100  R-US_M0805  [M0805]
R153  100  R-US_M0805  [M0805]
R154  100  R-US_M0805  [M0805]
R155  100  R-US_M0805  [M0805]
R156  100  R-US_M0805  [M0805]
R157  100  R-US_M0805  [M0805]
R158  100  R-US_M0805  [M0805]
R159  100  R-US_M0805  [M0805]
R161  100  R-US_M0805  [M0805]
R162  100  R-US_M0805  [M0805]
R163  100  R-US_M0805  [M0805]
R168  150  R-US_M0805  [M0805]
R169  150  R-US_M0805  [M0805]
R170  150  R-US_M0805  [M0805]
R171  150  R-US_M0805  [M0805]
R172  150  R-US_M0805  [M0805]
R173  150  R-US_M0805  [M0805]
R176  10K  R-US_R0603  [R0603]
S1  SWITCH-MOMENTARY-2-SMD-1101NE  [TACTILE-SWITCH-1101NE]
U$52  3.6V-NIMH-BATTERY  [3.6V-NIMH-BATTERY]
U$53  3.6V-NIMH-BATTERY  [3.6V-NIMH-BATTERY]
U$54  1X1  [1X1]
U$56  1X1  [1X1]
U$57  1X1  [1X1]
U$58  1X1  [1X1]
U$59  1X1  [1X1]
U$60  1X1  [1X1]
U$61  1X1  [1X1]
U$62  1X1  [1X1]
U$63  2X3  [2X3]
U$64  1X3  [1X3]
U$65  1X1  [1X1]
U$66  1X1  [1X1]
U$67  1X1  [1X1]
U$68  1X1  [1X1]
U$69  1X1  [1X1]
U$70  1X1  [1X1]
U$71  1X1  [1X1]
U$72  1X1  [1X1]
U$73  1X1  [1X1]
U$74  1X1  [1X1]
U$75  1X2  [1X2]

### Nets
CLOCK2: IC20.17(PB5(SCK)) IC22.11(SCK) IC23.11(SCK) IC24.11(SCK) U$63.5
DATA2: IC20.15(PB3(MOSI/OC2)) IC22.14(SER) U$63.6
GND: IC20.3(GND) IC20.5(GND) IC20.21(GND) IC22.13(G) IC23.13(G) IC24.13(G) S1.P$1 U$52.- U$53.- U$63.1 U$75.1 ; also sheet 1
LATCH2: IC20.14(PB2(SS/OC1B)) IC22.12(RCK) IC23.12(RCK) IC24.12(RCK)
MISO: IC20.16(PB4(MISO)) U$63.4
N$4: IC22.15(QA) R168.1
N$7: IC22.1(QB) R151.1
N$8: IC22.2(QC) R152.1
N$9: R168.2 U$54.1
N$10: R151.2 U$56.1
N$11: R152.2 U$57.1
N$12: R169.2 U$58.1
N$13: R153.2 U$59.1
N$14: R154.2 U$60.1
N$15: R170.2 U$61.1
N$16: R155.2 U$62.1
N$17: IC22.3(QD) R169.1
N$18: IC22.4(QE) R153.1
N$19: IC22.5(QF) R154.1
N$20: IC22.6(QG) R170.1
N$21: IC22.7(QH) R155.1
N$22: IC23.15(QA) R156.1
N$23: R156.2 U$65.1
N$24: R171.2 U$66.1
N$25: R157.2 U$67.1
N$26: R158.2 U$68.1
N$27: R172.2 U$69.1
N$28: R159.2 U$70.1
N$187: R161.2 U$71.1
N$188: R173.2 U$72.1
N$189: R162.2 U$73.1
N$190: R163.2 U$74.1
N$273: IC24.1(QB) R163.1
N$274: IC24.15(QA) R162.1
N$275: IC23.7(QH) R173.1
N$364: IC23.6(QG) R161.1
N$365: IC23.5(QF) R159.1
N$366: IC23.4(QE) R172.1
N$367: IC23.3(QD) R158.1
N$368: IC23.2(QC) R157.1
N$369: IC23.1(QB) R171.1
N$370: IC23.9(QH*) IC24.14(SER)
N$371: IC22.9(QH*) IC23.14(SER)
N$374: U$64.1 U$75.2
N$375: U$52.+ U$53.+ U$64.2
RESET2: IC20.29(PC6(/RESET)) R176.1 S1.P$2 U$63.3
VCC: IC20.4(VCC) IC20.6(VCC) IC20.18(AVCC) IC22.10(SCL) IC23.10(SCL) IC24.10(SCL) R176.2 U$63.2 U$64.3 ; also sheet 1
Unconnected: IC20.1(PD3(INT1)) IC20.2(PD4(XCK/T0)) IC20.7(PB6(XTAL1/TOSC1)) IC20.8(PB7(XTAL2/TOSC2)) IC20.9(PD5(T1)) IC20.10(PD6(AIN0)) IC20.11(PD7(AIN1)) IC20.12(PB0(ICP)) IC20.13(PB1(OC1A)) IC20.19(ADC6) IC20.20(AREF) IC20.22(ADC7) IC20.23(PC0(ADC0)) IC20.24(PC1(ADC1)) IC20.25(PC2(ADC2)) IC20.26(PC3(ADC3)) IC20.27(PC4(ADC4/SDA)) IC20.28(PC5(ADC5/SCL)) IC20.30(PD0(RXD)) IC20.31(PD1(TXD)) IC20.32(PD2(INT0)) IC24.2(QC) IC24.3(QD) IC24.4(QE) IC24.5(QF) IC24.6(QG) IC24.7(QH) IC24.9(QH*)

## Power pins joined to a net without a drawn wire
GND: IC1.8(GND) IC2.8(GND) IC3.8(GND) IC4.8(GND) IC5.8(GND) IC6.8(GND) IC7.8(GND) IC8.8(GND) IC9.8(GND) IC10.8(GND) IC11.8(GND) IC12.8(GND) IC13.8(GND) IC14.8(GND) IC15.8(GND) IC16.8(GND) IC17.8(GND) IC18.8(GND) IC19.8(GND) IC21.10(GND) IC22.8(GND) IC23.8(GND) IC24.8(GND)
VCC: IC1.16(VCC) IC2.16(VCC) IC3.16(VCC) IC4.16(VCC) IC5.16(VCC) IC6.16(VCC) IC7.16(VCC) IC8.16(VCC) IC9.16(VCC) IC10.16(VCC) IC11.16(VCC) IC12.16(VCC) IC13.16(VCC) IC14.16(VCC) IC15.16(VCC) IC16.16(VCC) IC17.16(VCC) IC18.16(VCC) IC19.16(VCC) IC21.20(VCC) IC22.16(VCC) IC23.16(VCC) IC24.16(VCC)

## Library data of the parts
C1 = resistor:CPOL-EU: POLARIZED CAPACITOR, European symbol
IC1-IC19 IC22-IC24 = 74xx-eu:74*595: 8-bit SHIFT REGISTER, output latch
IC20 = atmel:MEGA8: MICROCONTROLLER 8 Kbytes FLASH, 1 kbytes SRAM, 512 bytes EEPROM, USART, 6-channel 10 bit ADC, 2-channel 8 bit ADC Pin compatible with Atmega48, ATMega88, ATMega168 Source: avr.lbr; MPN: ATMEGA8-16AU; OC_FARNELL: 9171371; OC_NEWARK: 73M8863
IC21 = 74xx-us:74*245: Octal BUS TRANSCEIVER, 3-state
J1-J4 = con-molex:22-?-03: CONNECTOR wire to board 2.54 mm (.1 inch) pitch header; OC_FARNELL: unknown; OC_NEWARK: unknown
LED1-LED54 = adafruit:RGBLED_CA: RGB LED, common-anode 5MM Staggered pins 5mm Piranha package http://www.ladyada.net/library/pcb/eaglelibrary.html
R1-R163 R168-R173 R176 = resistor:R-US_: RESISTOR, American symbol
S1 = SparkFun-Electromechanical:SWITCH-MOMENTARY-2: Various NO switches- pushbuttons, reed, etc
U$1 = SparkFun-Boards:ARDUINO_PRO_MINI
U$2-U$51 U$64 = headers(2mm):1X3
U$52 U$53 = ggaqquay:3.6V-NIMH-BATTERY
U$54 U$56-U$62 U$65-U$74 = headers(2mm):1X1
U$55 = ggaqquay:LIMIT-SWITCH
U$63 = headers(2mm):2X3
U$75 = headers(2mm):1X2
